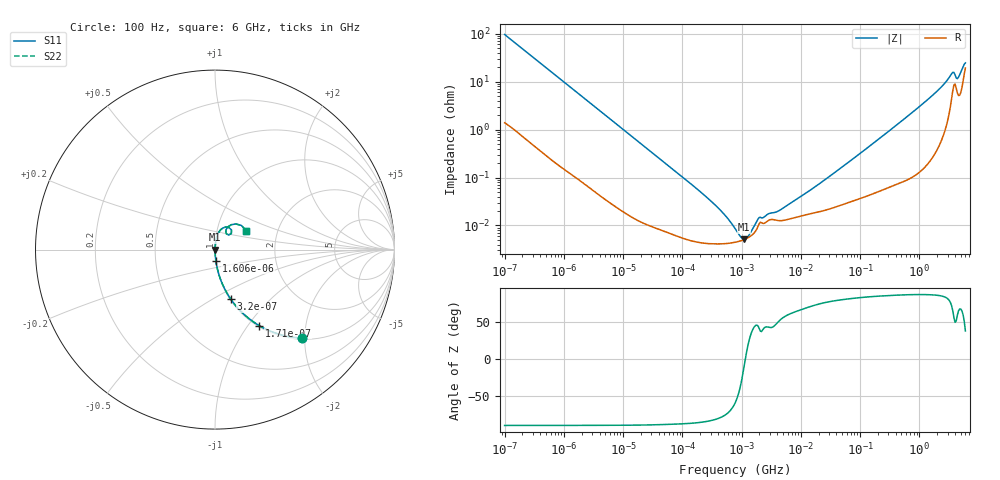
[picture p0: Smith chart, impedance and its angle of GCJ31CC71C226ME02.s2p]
!Murata Part Number: GCJ31CC71C226ME02
!These Parameters are Measured in Series Mode Connection
!Data Generated on Mar 13, 2026
!  o--ll--o
!Port1  Port2
!  o------o
!Operation Temp=25[degC], DC Bias Voltage=0[V]
!Freq. Start=100[Hz] Stop=6[GHz] 401[Steps]
# Hz S RI R 50
!Freq.(Hz) S11(Real) S11(Imag) S21(Real) S21(Imag) S12(Real) S12(Imag) S22(Real) S22(Imag)
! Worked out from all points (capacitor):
!   401 points, 100 Hz to 6 GHz, reference 50 ohm
!   read as one part in series: C = 16.4 uF near 109 Hz
!   lowest |Z| = 5.13 mohm at 1.108 MHz (marker M1)
!   series resonance near 1.155 MHz, so ESL is about 1.2 nH
!   S11 on the Smith chart (normalised r, x): 100 Hz: 1.03, -1.93; 171 Hz: 1.02, -1.13; 320 Hz: 1.01, -0.61; 1.606 kHz: 1.00, -0.12; 6 GHz: 1.39, +0.31
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100  0.4821 -0.4925  0.5179 0.4925  0.5179 0.4925  0.4821 -0.4925
171  0.2465 -0.4236  0.7535 0.4236  0.7535 0.4236  0.2465 -0.4236
320  0.0884 -0.2766  0.9116 0.2766  0.9116 0.2766  0.0884 -0.2766
686  0.0221 -0.1399  0.9779 0.1399  0.9779 0.1399  0.0221 -0.1399
1606  0.00477 -0.0613  0.9952 0.0613  0.9952 0.0613  0.00477 -0.0613
2008  0.00324 -0.0492  0.9968 0.0492  0.9968 0.0492  0.00324 -0.0492
40335  8.93e-05 -0.00253  0.9999 0.00253  0.9999 0.00253  8.93e-05 -0.00253
264476  4.2e-05 -0.000374  1 0.000374  1 0.000374  4.2e-05 -0.000374
452617  4.13e-05 -0.000196  1 0.000196  1 0.000196  4.13e-05 -0.000196
677235  4.32e-05 -0.000102  1 0.000102  1 0.000102  4.32e-05 -0.000102
774597  4.44e-05 -7.45e-05  1 7.45e-05  1 7.45e-05  4.44e-05 -7.45e-05
1108252  5.07e-05 -7.6e-06  0.9999 7.6e-06  0.9999 7.6e-06  5.07e-05 -7.6e-06
1585629  6.71e-05 6.06e-05  0.9999 -6.06e-05  0.9999 -6.06e-05  6.71e-05 6.06e-05
1983483  0.000109 9.76e-05  0.9999 -9.76e-05  0.9999 -9.76e-05  0.000109 9.76e-05
4440638  0.000125 0.000166  0.9999 -0.000166  0.9999 -0.000166  0.000125 0.000166
1.555665e7  0.000178 0.000552  0.9998 -0.000552  0.9998 -0.000552  0.000178 0.000552
3.124326e8  0.000713 0.00943  0.9993 -0.00943  0.9993 -0.00943  0.000713 0.00943
1.251881e9  0.00308 0.0377  0.9969 -0.0377  0.9969 -0.0377  0.00308 0.0377
2.562649e9  0.0148 0.0843  0.9852 -0.0843  0.9852 -0.0843  0.0148 0.0843
3.505958e9  0.0583 0.1254  0.9417 -0.1254  0.9417 -0.1254  0.0583 0.1254
4.586474e9  0.0597 0.1006  0.9403 -0.1006  0.9403 -0.1006  0.0597 0.1006
6e9  0.1752 0.1056  0.8248 -0.1056  0.8248 -0.1056  0.1752 0.1056
